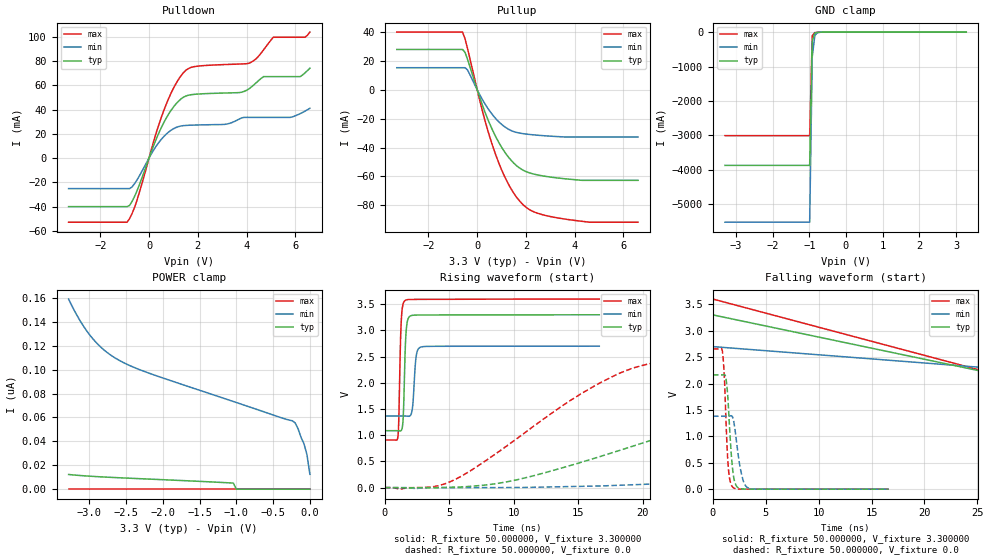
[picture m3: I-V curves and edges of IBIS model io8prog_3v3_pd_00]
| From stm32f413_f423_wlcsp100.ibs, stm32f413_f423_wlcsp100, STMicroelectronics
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|   Model io8prog_3v3_pd_00
[Model]  io8prog_3v3_pd_00
Model_type I/O
Polarity   Non-Inverting
Enable   Active-Low
Vinl =   0.990000V
Vinh =   2.310000V
Vmeas =  1.650000V
Cref =   100.000000nF
Rref =   1.000000k
Vref =   3.300000V
C_comp   2.665600pF   2.506300pF   2.859000pF
[Temperature Range]   25.000000   0.125000k   -40.000000
[Pullup Reference]   3.300000V   2.700000V   3.600000V
[Pulldown Reference]   0.0V   0.0V   0.0V
[POWER Clamp Reference]   3.300000V   2.700000V   3.600000V
[GND Clamp Reference]   0.0V   0.0V   0.0V
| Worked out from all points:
|   slope of the pulldown table from 0 to 0.495 V, typ, clamps not added: 20 ohm
|   slope of the pullup table from 0 to 0.495 V, typ, clamps not added: 21.7 ohm
|   GND clamp passes 1 mA (typ) near -0.57 V on its own axis
|   rising waveform, R_fixture 50.000000, V_fixture 3.300000: 20-80 % time 165ps typ, 208ps min, 154ps max; typ from 1.09 V to 3.3 V
|   rising waveform, R_fixture 50.000000, V_fixture 0.0: 20-80 % time 18.3ns typ, 43.3ns min, 9.75ns max; typ from 0 V to 2.16 V
|   falling waveform, R_fixture 50.000000, V_fixture 3.300000: 20-80 % time 31.6ns typ, 63.2ns min, 30.3ns max; typ from 3.3 V to 1.09 V
|   falling waveform, R_fixture 50.000000, V_fixture 0.0: 20-80 % time 421ps typ, 610ps min, 335ps max; typ from 2.16 V to 0 V
[Pulldown]
|Voltage   I(typ)   I(min)   I(max)
-3.3V     -40.11mA   -25.24mA   -52.93mA
-900mV    -40.11mA   -25.24mA   -52.93mA
-500mV    -27.39mA   -18.32mA   -35.21mA
600mV     29.01mA    17.61mA    38.88mA
1.1V      44.56mA    25.16mA    61.26mA
1.5V      51.11mA    26.89mA    72.21mA
3.1V      53.67mA    27.79mA    77.15mA
4.1V      57.1mA     33.57mA    78.25mA
4.7V      67.22mA    33.57mA    89.26mA
5.1V      67.22mA    33.57mA    99.69mA
6.2V      67.22mA    36.63mA    99.69mA
6.6V      74.18mA    41.08mA    104mA
[Pullup]
|Voltage   I(typ)   I(min)   I(max)
-3.3V     27.94mA    15.3mA     39.98mA
-600mV    27.94mA    15.3mA     39.98mA
-500mV    25.89mA    15.3mA     35.29mA
-400mV    21.3mA     13.82mA    28.75mA
300mV     -14.62mA   -9.248mA   -20.15mA
800mV     -33.8mA    -20.67mA   -46.89mA
1.1V      -42.41mA   -25.27mA   -59.19mA
1.4V      -49.01mA   -28.29mA   -68.91mA
2V        -56.64mA   -30.64mA   -81.32mA
2.6V      -59.37mA   -31.63mA   -86.15mA
3.9V      -62.11mA   -32.7mA    -90.24mA
6.6V      -62.7mA    -32.7mA    -91.7mA
[GND_clamp]
|Voltage   I(typ)   I(min)   I(max)
-3.3V     -3.872A    -5.523A    -3.009A
-990mV    -3.872A    -5.523A    -3.009A
-920mV    -262.2mA   -719.6mA   -104.3mA
-850mV    -25.2mA    -101mA     -13.09mA
-780mV    -6.971mA   -18.01mA   -7.205mA
3.28V     81.28uA    57.88uA    93.99uA
[POWER_clamp]
|Voltage   I(typ)   I(min)   I(max)
-3.28V    12.27nA    159nA      0A
-3.12V    11.41nA    140.5nA    0A
-2.96V    10.73nA    126.5nA    0A
-2.76V    10.05nA    114.5nA    0A
-2.56V    9.455nA    106.7nA    0A
-1.04V    5.085nA    73.31nA    0A
-1V       0A         72.48nA    0A
-240mV    0A         57.24nA    0A
-200mV    0A         55.42nA    0A
-80mV     0A         37.96nA    0A
-40mV     0A         28.96nA    0A
0V        0A         12.44nA    0A
[Ramp]
| variable   typ   min   max
dV/dt_r  1.29804/18.26314n   0.82812/43.29273n   1.59294/9.74051n
dV/dt_f  1.32738/17.43925n   0.79914/35.61971n   1.61393/10.83131n
R_load = 50.000000
[Rising Waveform]
R_fixture= 50.000000
V_fixture= 3.300000
V_fixture_min= 2.700000
V_fixture_max= 3.600000
|time   V(typ)   V(min)   V(max)
0s        1.087V     1.367V     909mV
1.034ns   1.086V     1.367V     995.3mV
1.268ns   1.088V     1.367V     3.118V
1.435ns   1.351V     1.367V     3.516V
1.568ns   2.494V     1.366V     3.571V
1.802ns   3.218V     1.362V     3.589V
2.135ns   3.288V     1.5V       3.592V
2.469ns   3.293V     2.553V     3.593V
2.803ns   3.294V     2.683V     3.593V
16.62ns   3.299V     2.699V     3.599V
[Rising Waveform]
R_fixture= 50.000000
V_fixture= 0.0
V_fixture_min= 0.0
V_fixture_max= 0.0
|time   V(typ)   V(min)   V(max)
0s        3.79nV     209.7nV    2.596nV
5.405ns   8.68mV     -130.6uV   149.2mV
10.21ns   147.9mV    2.258mV    931mV
19.22ns   791.6mV    54.52mV    2.282V
28.83ns   1.5V       185.2mV    2.579V
37.24ns   1.9V       352.3mV    2.631V
46.25ns   2.047V     550.8mV    2.647V
70.87ns   2.147V     1.029V     2.655V
99.1ns    2.161V     1.278V     2.655V
299.1ns   2.163V     1.38V      2.655V
[Falling Waveform]
R_fixture= 50.000000
V_fixture= 3.300000
V_fixture_min= 2.700000
V_fixture_max= 3.600000
|time   V(typ)   V(min)   V(max)
0s        3.299V     2.699V     3.599V
50.05ns   1.198V     1.923V     931.7mV
100.1ns   1.095V     1.445V     909.9mV
150.2ns   1.087V     1.384V     909.1mV
200.2ns   1.087V     1.371V     909mV
4.955us   1.087V     1.367V     909mV
[Falling Waveform]
R_fixture= 50.000000
V_fixture= 0.0
V_fixture_min= 0.0
V_fixture_max= 0.0
|time   V(typ)   V(min)   V(max)
0s        2.163V     1.38V      2.655V
900.9ps   2.164V     1.38V      2.607V
1.101ns   2.17V      1.38V      2.046V
1.201ns   2.13V      1.38V      1.486V
1.435ns   1.667V     1.381V     467.4mV
1.635ns   963mV      1.388V     144.5mV
1.902ns   313.9mV    1.339V     32.22mV
2.669ns   7.473mV    316mV      795.6uV
3.337ns   477.1uV    22.75mV    464.6uV
16.62ns   3.79nV     209.7nV    2.596nV
